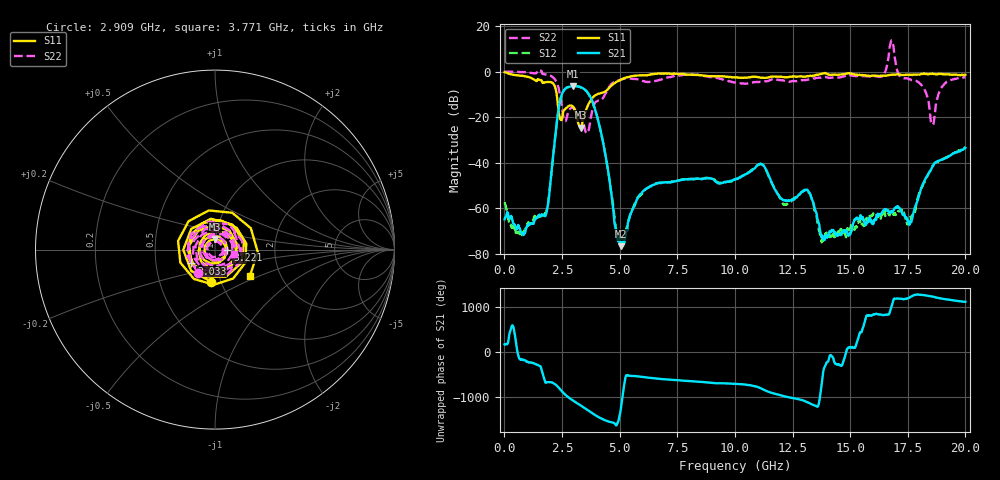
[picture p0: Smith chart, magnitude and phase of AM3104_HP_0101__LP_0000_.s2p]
!Created with skrf (http://scikit-rf.org).
# Hz S RI R 50.0
!freq ReS11 ImS11 ReS21 ImS21 ReS12 ImS12 ReS22 ImS22
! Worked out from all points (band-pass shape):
!   1601 points, 10 MHz to 20 GHz, reference 50 ohm
!   highest |S21| = -6.36 dB at 2.984 GHz (marker M1); lowest = -76.8 dB at 5.07 GHz (marker M2)
!   |S21| within 3 dB of the highest: 2.52 GHz to 3.623 GHz (1.104 GHz wide, 35.9 % of centre)
!   lowest |S11| = -24.6 dB at 3.321 GHz (marker M3), VSWR 1.12, Z = 49.6 + j5.86 ohm
!   |S11| at or under -10 dB: 2.269 GHz to 4.023 GHz (1.754 GHz wide, 55.7 % of centre)
!   |S22| runs from -27.2 to 13.7 dB; largest |S21 - S12| = 0.027
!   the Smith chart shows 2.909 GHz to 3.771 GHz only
!   S11 on the Smith chart (normalised r, x): 2.909 GHz: 0.90, -0.33; 3.033 GHz: 0.76, -0.12; 3.221 GHz: 1.15, -0.00; 3.771 GHz: 1.40, -0.44
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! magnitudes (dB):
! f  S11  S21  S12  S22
! 10 MHz  -0.3  -64.9  -57.5  -0.1
! 672.2 MHz  -1.8  -69.2  -71.5  -0.2
! 1.772 GHz  -4.7  -63.4  -62.4  -1.2
! 2.409 GHz  -20.5  -13.3  -13.3  -9.9
! 2.909 GHz  -14.9  -6.5  -6.6  -15.9
! 2.984 GHz  -15.6  -6.4  -6.4  -16.1
! 3.033 GHz  -16.4  -6.4  -6.4  -16.3
! 3.221 GHz  -23.2  -6.5  -6.6  -18.9
! 3.321 GHz  -24.6  -6.9  -7.0  -20.0
! 3.346 GHz  -24.3  -7.0  -7.1  -20.5
! 3.771 GHz  -12.3  -12.0  -12.1  -19.2
! 5.07 GHz  -3.5  -76.8  -72.8  -3.5
! 6.682 GHz  -0.9  -49.0  -49.0  -3.8
! 10.01 GHz  -2.6  -47.5  -47.8  -4.8
! 11.14 GHz  -2.7  -40.6  -40.8  -4.4
! 12.14 GHz  -2.4  -56.6  -58.4  -4.1
! 13.34 GHz  -2.0  -56.1  -55.9  -3.2
! 13.79 GHz  -0.8  -72.1  -74.6  -2.5
! 16.68 GHz  -1.6  -61.6  -62.8  7.2
! 17.6 GHz  -1.5  -66.2  -65.2  -3.4
! 18.56 GHz  -0.9  -42.0  -41.6  -23.2
! 20 GHz  -1.4  -33.6  -33.3  -2.5
